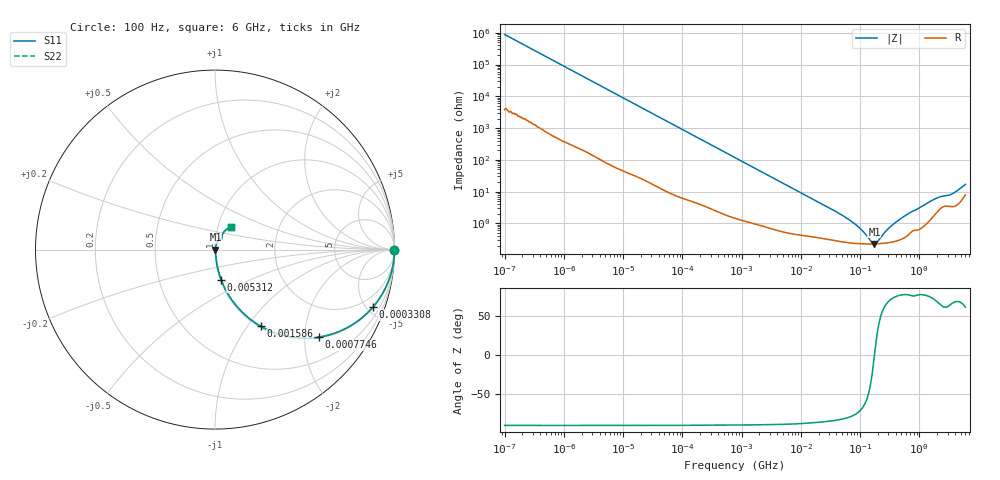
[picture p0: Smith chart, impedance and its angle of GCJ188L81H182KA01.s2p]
!Murata Part Number: GCJ188L81H182KA01
!These Parameters are Measured in Series Mode Connection
!Data Generated on Mar 13, 2026
!  o--ll--o
!Port1  Port2
!  o------o
!Operation Temp=25[degC], DC Bias Voltage=0[V]
!Freq. Start=100[Hz] Stop=6[GHz] 401[Steps]
# Hz S RI R 50
!Freq.(Hz) S11(Real) S11(Imag) S21(Real) S21(Imag) S12(Real) S12(Imag) S22(Real) S22(Imag)
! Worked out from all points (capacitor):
!   401 points, 100 Hz to 6 GHz, reference 50 ohm
!   read as one part in series: C = 1.8 nF near 109 Hz
!   lowest |Z| = 227 mohm at 174.6 MHz (marker M1)
!   series resonance near 174.8 MHz, so ESL is about 460 pH
!   S11 on the Smith chart (normalised r, x): 100 Hz: open; 330.8 kHz: 1.05, -5.49; 774.6 kHz: 1.03, -2.36; 1.586 MHz: 1.02, -1.16; 5.312 MHz: 1.01, -0.35; 6 GHz: 1.16, +0.30
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100  1 -0.000113  5e-07 0.000113  5e-07 0.000113  1 -0.000113
2008  1 -0.00225  1.56e-05 0.00225  1.56e-05 0.00225  1 -0.00225
40335  0.9977 -0.0447  0.00226 0.0447  0.00226 0.0447  0.9977 -0.0447
123542  0.9807 -0.1339  0.0193 0.1339  0.0193 0.1339  0.9807 -0.1339
330837  0.8806 -0.3194  0.1194 0.3194  0.1194 0.3194  0.8806 -0.3194
495019  0.7696 -0.4158  0.2304 0.4158  0.2304 0.4158  0.7696 -0.4158
774597  0.5804 -0.4874  0.4196 0.4874  0.4196 0.4874  0.5804 -0.4874
1585629  0.2545 -0.427  0.7455 0.427  0.7455 0.427  0.2545 -0.427
2713602  0.1087 -0.3006  0.8913 0.3006  0.8913 0.3006  0.1087 -0.3006
5311619  0.0343 -0.1676  0.9657 0.1676  0.9657 0.1676  0.0343 -0.1676
1.555665e7  0.00732 -0.0593  0.9927 0.0593  0.9927 0.0593  0.00732 -0.0593
7.129496e7  0.00253 -0.0114  0.9975 0.0114  0.9975 0.0114  0.00253 -0.0114
1.066761e8  0.00231 -0.00574  0.9977 0.00574  0.9977 0.00574  0.00231 -0.00574
1.596157e8  0.00226 -0.00102  0.9977 0.00102  0.9977 0.00102  0.00226 -0.00102
1.745687e8  0.00227 -1.26e-05  0.9977 1.26e-05  0.9977 1.26e-05  0.00227 -1.26e-05
1.996653e8  0.00229 0.0015  0.9977 -0.0015  0.9977 -0.0015  0.00229 0.0015
3.124326e8  0.00254 0.00691  0.9975 -0.00691  0.9975 -0.00691  0.00254 0.00691
6.11557e8  0.00424 0.0183  0.9958 -0.0183  0.9958 -0.0183  0.00424 0.0183
1.497423e9  0.0142 0.0453  0.9858 -0.0453  0.9858 -0.0453  0.0142 0.0453
2.142435e9  0.0291 0.0582  0.9709 -0.0582  0.9709 -0.0582  0.0291 0.0582
3.505958e9  0.0377 0.0709  0.9623 -0.0709  0.9623 -0.0709  0.0377 0.0709
6e9  0.0912 0.1251  0.9088 -0.1251  0.9088 -0.1251  0.0912 0.1251
